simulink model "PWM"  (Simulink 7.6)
settings: Solver=ode15s  StartTime=0.0  StopTime=10  RelTol=1e-3
StopFcn:
  | load pwm.mat
  | plot(x(1,:),x(2,:),x(1,:),x(3,:))
  | axis([0 10 -0.2 4.2])
  | grid
undefined symbols (not defined in the file or in its folder): sigbuilder_block
libraries: fl_lib x5, nesl_utility x3, elec_lib x1

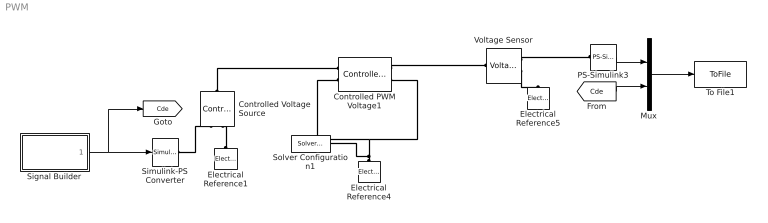
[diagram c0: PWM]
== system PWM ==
  Controlled PWM Voltage1 : elec_lib/Actuators & Drivers/Drivers/Controlled PWM Voltage  DialogController=NetworkEngine.DynNeDlgSource  SystemSampleTime=-1  F=1 Hz  Vmin=0 V  Vmax=5 V  Vm=2.5 V  pwm_or_av=1  current_Log=off  voltage_Log=off  power_Log=off  LocalVarNames=|current|voltage|power  LocalVarDescs=|Load current (A)|Load voltage (V)|Load power (W)  LocalVarLogging=[0 0 0]
  Controlled Voltage Source : fl_lib/Electrical/Electrical Sources/Controlled Voltage Source  DialogController=NetworkEngine.DynNeDlgSource  SystemSampleTime=-1  i_Log=off  v_Log=off  LocalVarNames=|i|v  LocalVarDescs=|i|v  LocalVarLogging=[0 0]
  Electrical Reference1 : fl_lib/Electrical/Electrical Elements/Electrical Reference  DialogController=NetworkEngine.DynNeDlgSource  SystemSampleTime=-1  i_Log=off  LocalVarNames=|i  LocalVarDescs=|i  LocalVarLogging=[]
  Electrical Reference4 : fl_lib/Electrical/Electrical Elements/Electrical Reference  DialogController=NetworkEngine.DynNeDlgSource  SystemSampleTime=-1  i_Log=off  LocalVarNames=|i  LocalVarDescs=|i  LocalVarLogging=[]
  Electrical Reference5 : fl_lib/Electrical/Electrical Elements/Electrical Reference  DialogController=NetworkEngine.DynNeDlgSource  SystemSampleTime=-1  i_Log=off  LocalVarNames=|i  LocalVarDescs=|i  LocalVarLogging=[]
  Mux : Mux  Inputs=2
  PS-Simulink3 : nesl_utility/PS-Simulink Converter  DialogController=NetworkEngine.DynNeUtilDlgSource  SystemSampleTime=-1  PhysicalDomain=network_engine_domain  LeftPortType=input  RightPortType=output  SubClassName=ps_output  Unit=V  AffineConversion=off
  Signal Builder : Subsystem  Tag=STV Subsys  LoadFcn=sigbuilder_block('load');  StartFcn=sigbuilder_block('start');  StopFcn=sigbuilder_block('stop');  ClipboardFcn=sigbuilder_block('clipboard');
  Simulink-PS Converter : nesl_utility/Simulink-PS Converter  DialogController=NetworkEngine.DynNeUtilDlgSource  SystemSampleTime=-1  PhysicalDomain=network_engine_domain  LeftPortType=input  RightPortType=output  SubClassName=ps_input  Unit=1  AffineConversion=off  InputFilterTimeConstant=.001  UdotUserProvided=0
  Solver Configuration1 : nesl_utility/Solver Configuration  DialogController=NetworkEngine.DynNeUtilDlgSource  SystemSampleTime=-1  PhysicalDomain=network_engine_domain  LeftPortType=input  RightPortType=generic  SubClassName=solver  Accelerate=off  Profile=off  ResidualTolerance=1e-9  MaxNonlinIter=12  MaxModeIter=2  DoFixedCost=off  UseLocalSampling=off  DoDC=off  LinearAlgebra=Full  LocalSolverSampleTime=.001  LocalSolverChoice=NE_BACKWARD_EULER_ADVANCER  UseLocalSolver=off
  To File1 : ToFile  Filename=pwm.mat  MatrixName=x
  Voltage Sensor : fl_lib/Electrical/Electrical Sensors/Voltage Sensor  DialogController=NetworkEngine.DynNeDlgSource  SystemSampleTime=-1  i1_Log=off  v1_Log=off  LocalVarNames=|i1|v1  LocalVarDescs=|i1|v1  LocalVarLogging=[]
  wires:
  Signal Builder/1(Signal 1) -> Simulink-PS Converter/1, [Cde]
  PS-Simulink3/1 -> Mux/1
  Mux/1 -> To File1/1
  [Cde] -> Mux/2
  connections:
  Electrical Reference4/LConn1 -- Controlled PWM Voltage1/RConn2 -- Controlled PWM Voltage1/LConn2 -- Solver Configuration1/RConn1
  Controlled PWM Voltage1/RConn1 -- Voltage Sensor/LConn1
  Voltage Sensor/RConn1 -- PS-Simulink3/LConn1
  Voltage Sensor/RConn2 -- Electrical Reference5/LConn1
  Controlled Voltage Source/LConn1 -- Controlled PWM Voltage1/LConn1
  Electrical Reference1/LConn1 -- Controlled Voltage Source/RConn2
  Simulink-PS Converter/RConn1 -- Controlled Voltage Source/RConn1

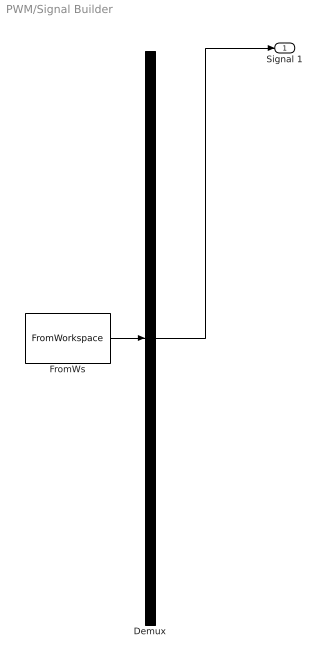
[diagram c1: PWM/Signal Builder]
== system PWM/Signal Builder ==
  Demux : Demux  Tag=STV Demux  Outputs=1
  FromWs : FromWorkspace  Tag=STV FromWs  VariableName=tuvar  SampleTime=0  SigBuilderData=DataTag0  VnvData=DataTag1
  Signal 1 : Outport  Tag=STV Outport
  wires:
  Demux/1 -> Signal 1/1
  FromWs/1 -> Demux/1
